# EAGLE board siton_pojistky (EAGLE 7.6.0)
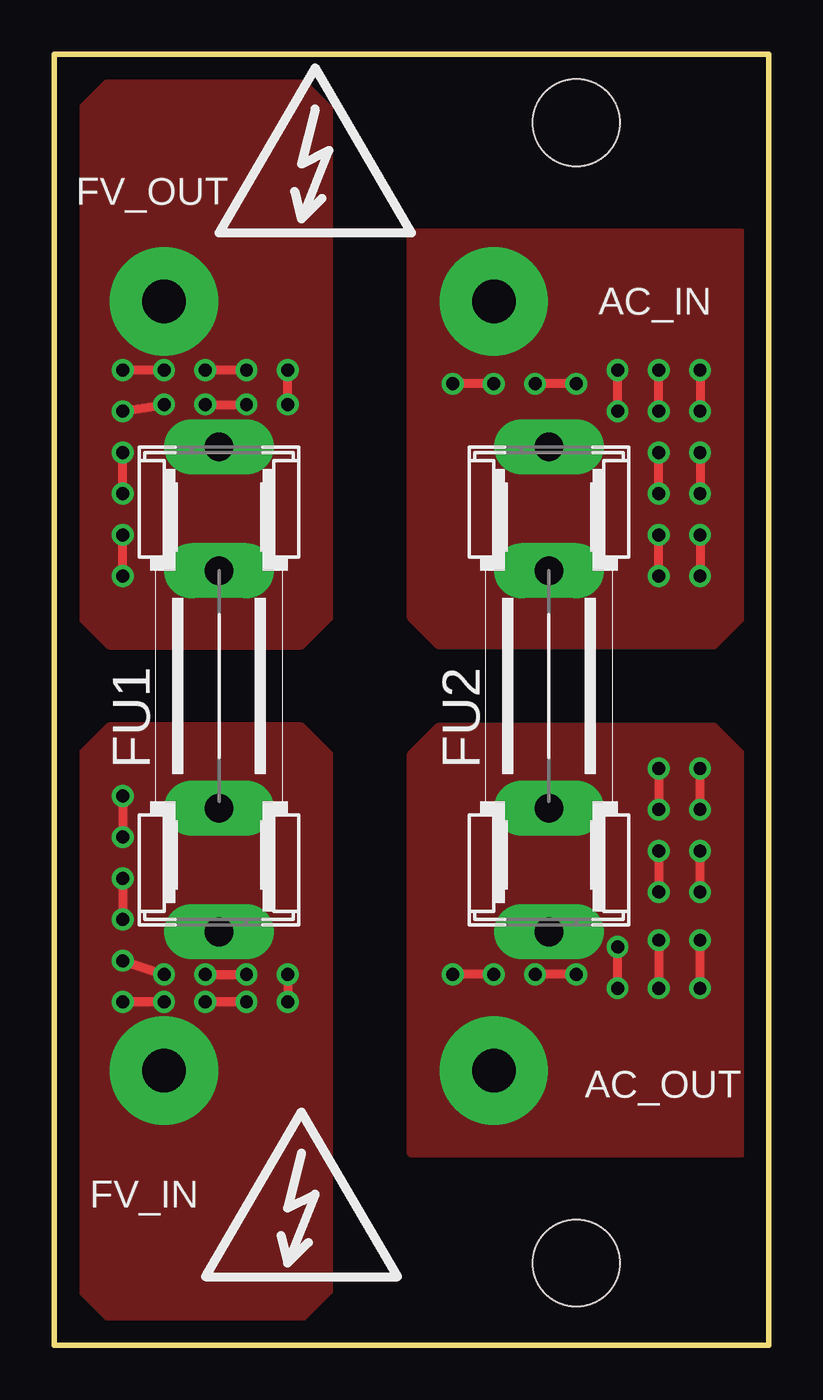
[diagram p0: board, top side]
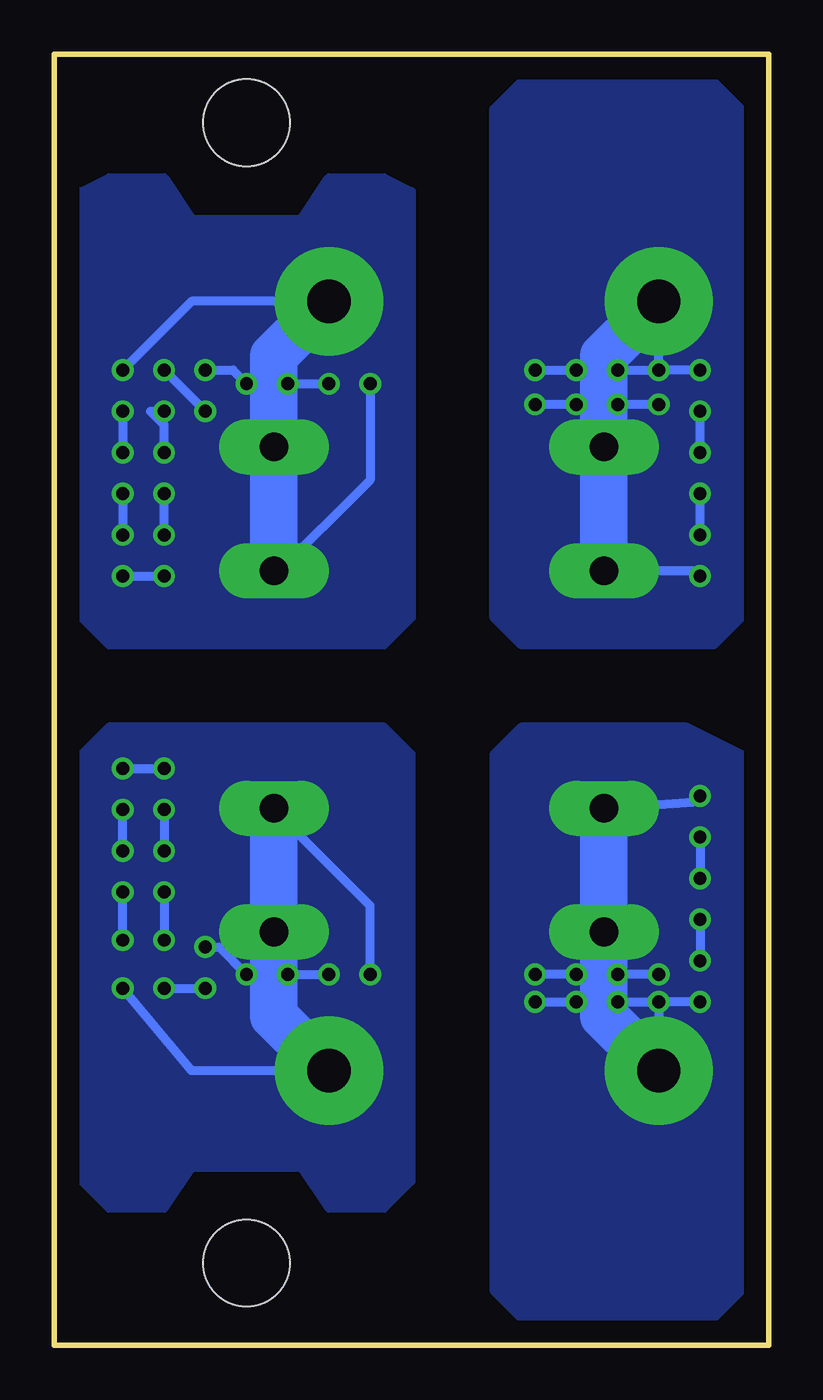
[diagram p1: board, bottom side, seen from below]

Size 33.02 x 59.69 mm. Coordinates in mm from the lower left corner, seen from the top.
Outline: 0,0 33.02,0 33.02,59.69 0,59.69 0,0
Copper layers (1*16): Top 0.035mm / dielectric 1.5mm / Bottom 0.035mm
Design rules "default": minimum track width 10mil, minimum drill 24mil, track to track 8mil, track to pad 8mil, pad to pad 8mil, via to via 8mil, smd to smd 8mil, copper to edge 40mil, drill to drill 8mil, minimum pad ring 10mil, minimum via ring 8mil, stop-mask expansion 4mil, vias tented up to drill 0mil, thermal gap 10mil
Holes 4 mm at 24.13,3.81 24.13,56.52

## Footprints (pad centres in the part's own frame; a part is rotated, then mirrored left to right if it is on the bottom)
LSP13 = drill 2 pad 5: MP 0,0
SHK20L = drill 1.321 pad 2.54 long: 1A -11.367,0; 1B -5.652,0; 2A 11.049,0; 2B 5.334,0

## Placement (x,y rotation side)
AC_IN  [LSP13]  20.32,48.26 0 top
AC_OUT  [LSP13]  20.32,12.7 0 top
FU1  12.5A  [SHK20L]  7.62,30.48 90 top
FU2  12.5A  [SHK20L]  22.86,30.48 90 top
FV_IN  [LSP13]  5.08,12.7 0 top
FV_OUT  [LSP13]  5.08,48.26 0 top

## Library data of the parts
AC_IN AC_OUT FV_IN FV_OUT = 12moje
FU1 FU2 = fuse2

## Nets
AC1: AC_IN.MP FU2.2A FU2.2B
AC2: AC_OUT.MP FU2.1A FU2.1B
FV1: FU1.2A FU1.2B FV_OUT.MP
VF2: FU1.1A FU1.1B FV_IN.MP

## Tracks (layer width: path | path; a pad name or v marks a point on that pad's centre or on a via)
AC1  (via drill 0.6)
  Top 0.406: FU2.2B 22.86,35.56 | v29.84,45.09 v29.84,43.18 | v29.84,41.27 v29.84,39.37 | v29.84,37.47 v29.84,35.56 | v27.94,35.56 v27.94,37.47 | v27.94,39.37 v27.94,41.27 | v27.94,43.18 v27.94,45.09 | v26.04,43.18 v26.04,45.09 | v24.13,44.45 v22.23,44.45 | v20.32,44.45 v18.41,44.45
  Bottom 0.406: AC_IN.MP 26.67,48.26 v29.84,45.09 | v29.84,43.18 v29.84,41.27 | v29.84,39.37 v29.84,37.47 | v29.84,35.56 v27.94,35.56 | v27.94,37.47 v27.94,39.37 | v27.94,41.27 27.94,42.55 28.57,43.18 v27.94,43.18 | v27.94,45.09 v26.04,43.18 | v26.04,45.09 24.77,45.09 v24.13,44.45 | v22.23,44.45 v20.32,44.45 | v18.41,44.45 18.41,40.01 22.86,35.56
  Bottom 2.184: FU2.2B FU2.2A 22.86,45.72 AC_IN.MP
  pour Bottom (no thermals): 17.78,32.38 30.48,32.38 31.75,33.66 31.75,53.34 30.48,53.98 27.94,53.98 26.67,52.07 21.59,52.07 20.32,53.98 17.78,53.98 16.51,53.34 16.51,33.66
  pour Top (no thermals): 30.48,32.38 17.78,32.38 16.51,33.66 16.51,51.44 31.75,51.44 31.75,33.66
AC2  (via drill 0.6)
  Top 0.406: v29.84,16.51 v29.84,18.73 | v29.84,20.95 v29.84,22.86 | v29.84,24.77 v29.84,26.67 | v27.94,26.67 v27.94,24.77 | v27.94,22.86 v27.94,20.95 | v27.94,18.73 v27.94,16.51 | v26.04,16.51 v26.04,18.41 | v24.13,17.14 v22.23,17.14 | v20.32,17.14 v18.41,17.14
  Bottom 0.406: AC_OUT.MP 26.67,12.7 v29.84,16.51 | v29.84,18.73 v29.84,20.95 | v29.84,22.86 v29.84,24.77 | v29.84,26.67 v27.94,26.67 | v27.94,24.77 v27.94,22.86 | v27.94,20.95 v27.94,18.73 | v27.94,16.51 v26.04,16.51 | v26.04,18.41 25.4,18.41 v24.13,17.14 | v22.23,17.14 v20.32,17.14 | v18.41,17.14 18.41,20.32 22.86,24.77
  Bottom 2.184: FU2.1B 22.86,24.77 FU2.1A 22.86,15.24 AC_OUT.MP
  pour Bottom (no thermals): 17.78,28.57 30.48,28.57 31.75,27.3 31.75,7.62 30.48,6.35 27.94,6.35 26.67,8.26 21.59,8.26 20.32,6.35 17.78,6.35 16.51,7.62 16.51,27.3
  pour Top (no thermals): 17.78,28.57 30.48,28.57 31.75,27.3 31.75,8.89 16.51,8.89 16.51,27.3
FV1  (via drill 0.6)
  Top 0.406: v3.17,35.56 v3.17,37.47 | v3.17,39.37 v3.17,41.27 | v3.17,43.18 v5.08,43.5 | v6.99,43.5 v8.89,43.5 | v10.79,43.5 v10.79,45.09 | v8.89,45.09 v6.99,45.09 | v5.08,45.09 v3.17,45.09
  Bottom 0.406: FU1.2B 3.17,35.81 v3.17,35.56 | v3.17,37.47 v3.17,39.37 | v3.17,41.27 v3.17,43.18 | v5.08,43.5 v6.99,43.5 | v8.89,43.5 v10.79,43.5 | v10.79,45.09 v8.89,45.09 | v6.99,45.09 v5.08,45.09 | v3.17,45.09 v5.08,45.09 | v5.08,45.09 FV_OUT.MP
  Bottom 2.184: FU1.2B FU1.2A 7.62,45.72 FV_OUT.MP
  pour Bottom (no thermals): 2.54,32.38 11.43,32.38 12.7,33.66 12.7,57.15 11.43,58.42 2.54,58.42 1.27,57.15 1.27,33.66
  pour Top (no thermals): 2.54,32.38 11.43,32.38 12.7,33.66 12.7,57.15 11.43,58.42 2.54,58.42 1.27,57.15 1.27,33.66
VF2  (via drill 0.6)
  Top 0.406: v3.17,25.4 v3.17,23.5 | v3.17,21.59 v3.17,19.68 | v3.17,17.78 v5.08,17.14 | v6.99,17.14 v8.89,17.14 | v10.79,17.14 v10.79,15.88 | v8.89,15.88 v6.99,15.88 | v5.08,15.88 v3.17,15.88
  Bottom 0.406: FU1.1B 3.17,25.15 v3.17,25.4 | v3.17,23.5 v3.17,21.59 | v3.17,19.68 v3.17,17.78 | v5.08,17.14 v6.99,17.14 | v8.89,17.14 v10.79,17.14 | v10.79,15.88 v8.89,15.88 | v6.99,15.88 v5.08,15.88 | v3.17,15.88 v5.08,15.88 | v5.08,15.88 FV_IN.MP
  Bottom 2.184: FU1.1B FU1.1A 7.62,15.24 FV_IN.MP
  pour Bottom (no thermals): 3.81,28.57 11.43,28.57 12.7,27.3 12.7,2.54 11.43,1.27 2.54,1.27 1.27,2.54 1.27,27.3
  pour Top (no thermals): 11.43,28.57 2.54,28.57 1.27,27.3 1.27,2.54 2.54,1.27 11.43,1.27 12.7,2.54 12.7,27.3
